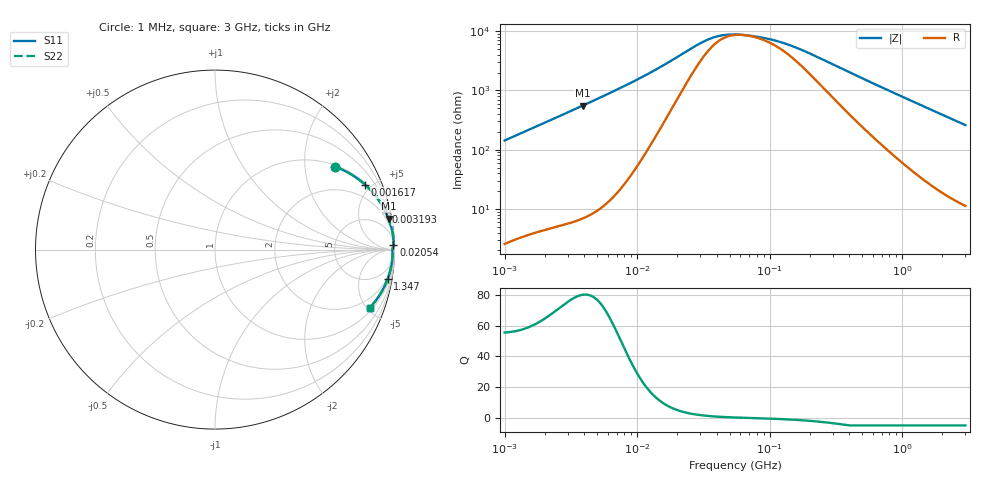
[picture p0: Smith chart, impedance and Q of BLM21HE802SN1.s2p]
! BLM21HE802SN1
# Hz S RI R 50
!Freq.(Hz) S11(Real) S11(Imag) S21(Real) S21(Imag) S12(Real) S12(Imag) S22(Real) S22(Imag)
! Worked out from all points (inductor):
!   401 points, 1 MHz to 3 GHz, reference 50 ohm
!   read as one part in series: L = 22.7 uH near 1.041 MHz
!   highest Q = 80.2 at 3.9 MHz (marker M1), where L = 22.7 uH
!   self-resonance near 63.31 MHz
!   S11 on the Smith chart (normalised r, x): 1 MHz: 1.05, +2.86; 1.617 MHz: 1.08, +4.60; 3.193 MHz: 1.12, +9.09; 20.54 MHz: 17, +74; 1.347 GHz: 2, -12; 3 GHz: 1.23, -5.20
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1000000  0.669 0.4617  0.331 -0.4617  0.331 -0.4617  0.669 0.4617
1616692  0.8371 0.361  0.1629 -0.361  0.1629 -0.361  0.8371 0.361
2226959  0.9058 0.2848  0.0942 -0.2848  0.0942 -0.2848  0.9058 0.2848
3192880  0.9514 0.2087  0.0486 -0.2087  0.0486 -0.2087  0.9514 0.2087
3823119  0.9655 0.1765  0.0345 -0.1765  0.0345 -0.1765  0.9655 0.1765
3900413  0.9668 0.1732  0.0332 -0.1732  0.0332 -0.1732  0.9668 0.1732
8179831  0.9914 0.0814  0.00856 -0.0814  0.00856 -0.0814  0.9914 0.0814
1.461624e7  0.9947 0.041  0.00527 -0.041  0.00527 -0.041  0.9947 0.041
2.054061e7  0.9939 0.0256  0.00609 -0.0256  0.00609 -0.0256  0.9939 0.0256
2.886629e7  0.9921 0.0146  0.00788 -0.0146  0.00788 -0.0146  0.9921 0.0146
3.597591e7  0.9908 0.00939  0.00915 -0.00939  0.00915 -0.00939  0.9908 0.00939
4.394807e7  0.9898 0.00557  0.0102 -0.00557  0.0102 -0.00557  0.9898 0.00557
5.477226e7  0.989 0.00207  0.011 -0.00207  0.011 -0.00207  0.989 0.00207
7.697298e7  0.9882 -0.00269  0.0118 0.00269  0.0118 0.00269  0.9882 -0.00269
1.081723e8  0.9882 -0.0077  0.0118 0.0077  0.0118 0.0077  0.9882 -0.0077
1.460522e8  0.9886 -0.0132  0.0114 0.0132  0.0114 0.0132  0.9886 -0.0132
2.094008e8  0.989 -0.022  0.011 0.022  0.011 0.022  0.989 -0.022
4.391493e8  0.9878 -0.0525  0.0122 0.0525  0.0122 0.0525  0.9878 -0.0525
8.005644e8  0.9808 -0.0982  0.0192 0.0982  0.0192 0.0982  0.9808 -0.0982
1.347129e9  0.9619 -0.1634  0.0381 0.1634  0.0381 0.1634  0.9619 -0.1634
2.050964e9  0.9257 -0.2395  0.0743 0.2395  0.0743 0.2395  0.9257 -0.2395
3e9  0.861 -0.3249  0.139 0.3249  0.139 0.3249  0.861 -0.3249
